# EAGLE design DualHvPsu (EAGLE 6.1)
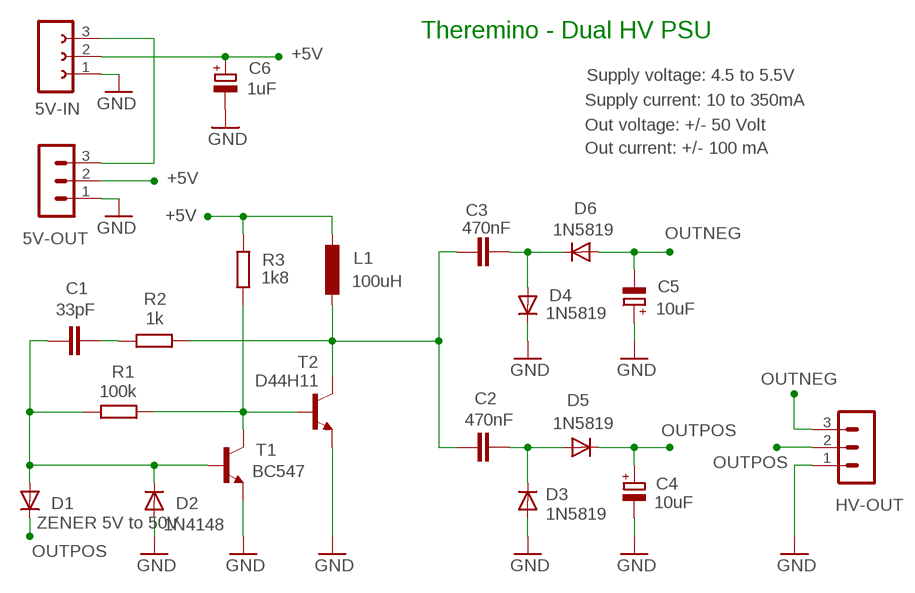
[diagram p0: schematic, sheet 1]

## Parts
5V-IN  FE03-1"  [FE03-1]
5V-OUT  MA03-1N  [MA03-1]
C1  33pF  C-EU025-024X044  [C025-024X044]
C2  470nF  C-EU050-024X044  [C050-024X044]
C3  470nF  C-EU050-024X044  [C050-024X044]
C4  10uF  CPOL-EUE2.5-5  [E2,5-5]
C5  10uF  CPOL-EUE2.5-5  [E2,5-5]
C6  1uF  CPOL-EUE2.5-5  [E2,5-5]
D1  ZENER 5V to 50V  DIODE-DO34-7  [DO34-7]
D2  1N4148  DIODE-DO34-7  [DO34-7]
D3  1N5819  DIODE-DO34-7  [DO34-7]
D4  1N5819  DIODE-DO34-7  [DO34-7]
D5  1N5819  DIODE-DO34-7  [DO34-7]
D6  1N5819  DIODE-DO34-7  [DO34-7]
HV-OUT  MA03-1N  [MA03-1]
L1  100uH  INDUCTORL_VERT_508  [L_VERT_508]
R1  100k  R-EU_0204/7  [0204/7]
R2  1k  R-EU_0204/7  [0204/7]
R3  1k8  R-EU_0204/7  [0204/7]
T1  BC547  -NPN-TO92-CBE  [TO92-CBE]
T2  D44H11  -NPN-TO220  [TO220]

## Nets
+5V: 5V-IN.2 5V-OUT.2 C6.+ L1.+ R3.2
GND: 5V-IN.1 5V-OUT.1 C4.- C5.+ C6.- D2.A D3.A D4.C HV-OUT.1 T1.E T2.3(E)
N$1: C1.1 D1.A D2.C R1.2 T1.B
N$2: C1.2 R2.2
N$3: 5V-IN.3 5V-OUT.3
N$4: C2.1 D3.C D5.A
N$5: C3.2 D4.A D6.C
N$12: C2.2 C3.1 L1.- R2.1 T2.2(C)
N$26: R1.1 R3.1 T1.C T2.1(B)
OUTNEG: C5.- D6.A HV-OUT.3
OUTPOS: C4.+ D1.C D5.C HV-OUT.2

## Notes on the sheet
- Theremino - Dual HV PSU
- Supply voltage: 4.5 to 5.5V
- Supply current: 10 to 350mA
- Out voltage: +/- 50 Volt
- Out current: +/- 100 mA

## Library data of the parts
5V-IN = 02-con-lsta-F:FE03-1: FEMALE HEADER
5V-OUT HV-OUT = 03-con-lstb-M:MA03-1: PIN HEADER
C1-C3 = 00-LIVIO:C-EU: CAPACITOR, European symbol
C4-C6 = 00-LIVIO:CPOL-EU: POLARIZED CAPACITOR, European symbol
D1-D6 = 00-LIVIO:DIODE-: DIODE
L1 = 00-LIVIO:INDUCTOR
R1-R3 = 00-LIVIO:R-EU_: RESISTOR, European symbol
T1 T2 = 00-LIVIO:*-NPN-: NPN Transistror

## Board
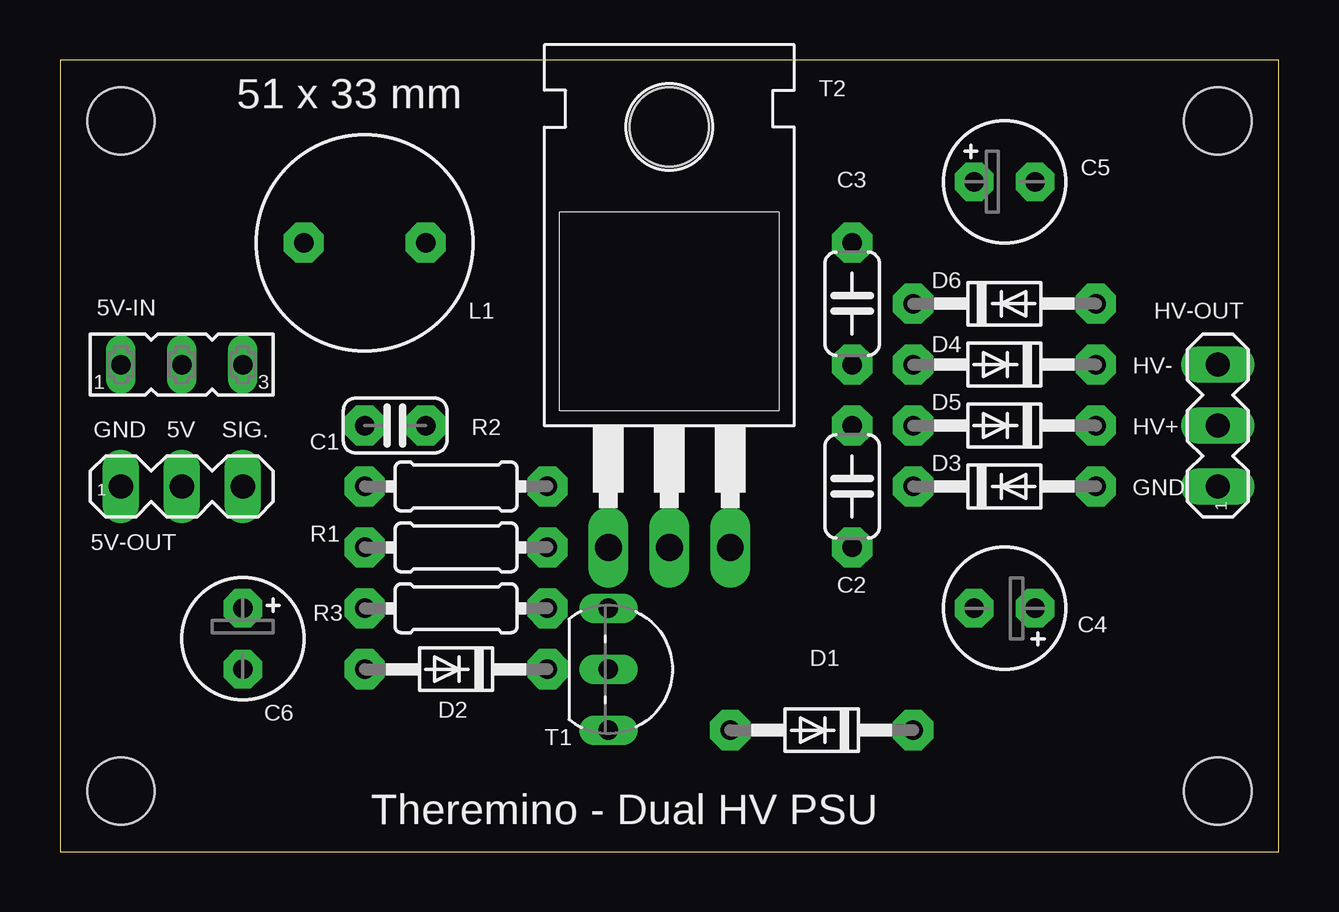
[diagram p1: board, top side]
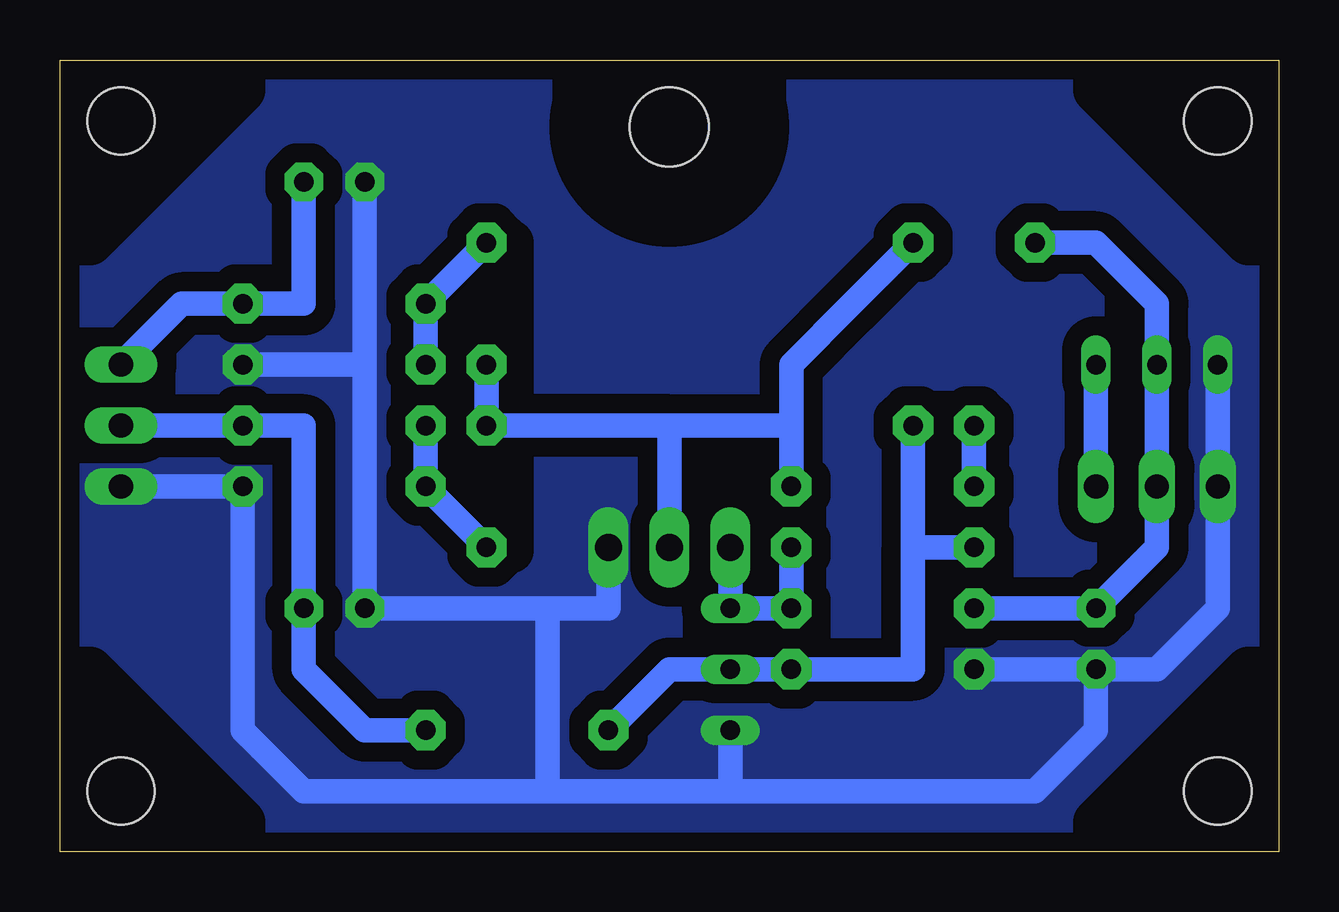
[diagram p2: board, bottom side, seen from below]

Size 50.8 x 33.02 mm. Coordinates in mm from the lower left corner, seen from the top.
Outline: 50.8,33.02 0,33.02 0,0 50.8,0 50.8,33.02
Copper layers (1*16): Top 0.035mm / dielectric 1.5mm / Bottom 0.035mm
Design rules: minimum track width 10mil, minimum drill 0.6mm, track to track 8mil, track to pad 8mil, pad to pad 8mil, via to via 8mil, smd to smd 8mil, copper to edge 31mil, drill to drill 8mil, minimum pad ring 5mil, minimum via ring 8mil, stop-mask expansion 4mil, vias tented up to drill 0mil, thermal gap 41mil
Holes 2.8 mm at 2.54,30.48 48.26,30.48 2.54,2.54 48.26,2.54
bRestrict: 10 lines

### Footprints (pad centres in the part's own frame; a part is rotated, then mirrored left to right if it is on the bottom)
FE03-1 = drill 0.813 long: 1 -2.54,0; 2 0,0; 3 2.54,0
MA03-1 = drill 1.016 long: 1 -2.54,0; 2 0,0; 3 2.54,0
C025-024X044 = drill 0.813 pad 1.676 octagon: 1 -1.27,0; 2 1.27,0
C050-024X044 = drill 0.813 pad 1.676 octagon: 1 -2.54,0; 2 2.54,0
E2,5-5 = drill 0.813 pad 1.6 octagon: + -1.27,0; - 1.27,0
DO34-7 = drill 0.813 pad 1.676 octagon: A 3.81,0; C -3.81,0
L_VERT_508 = drill 0.813 pad 1.676 octagon: + -2.54,0; - 2.54,0
0204/7 = drill 0.813 pad 1.676 octagon: 1 -3.81,0; 2 3.81,0
TO92-CBE = drill 0.813 long: B 0,0; C -2.54,0; E 2.54,0
TO220 = drill 1.118 long: 1 -2.54,-6.35; 2 0,-6.35; 3 2.54,-6.35 | hole 3.302: 0,11.176

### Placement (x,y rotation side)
5V-IN  5.08,20.32 0 top
5V-OUT  5.08,15.24 0 top
C1  13.97,17.78 180 top
C2  33.02,15.24 90 top
C3  33.02,22.86 90 top
C4  39.37,10.16 180 top
C5  39.37,27.94 0 top
C6  7.62,8.89 270 top
D1  31.75,5.08 180 top
D2  16.51,7.62 180 top
D3  39.37,15.24 0 top
D4  39.37,20.32 180 top
D5  39.37,17.78 180 top
D6  39.37,22.86 0 top
HV-OUT  48.26,17.78 90 top
L1  12.7,25.4 0 top
R1  16.51,12.7 180 top
R2  16.51,15.24 180 top
R3  16.51,10.16 180 top
T1  22.86,7.62 270 top
T2  25.4,19.05 0 top

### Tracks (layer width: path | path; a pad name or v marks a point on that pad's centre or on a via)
+5V
  Bottom 1.016: 5V-IN.2 5V-OUT.2 | 5V-OUT.2 5V-IN.2 | 5V-IN.2 5.08,22.86 7.62,25.4 L1.+ | R3.2 C6.+ 5.08,12.7 5V-OUT.2
GND
  Bottom 1.016: 22.86,2.54 20.32,2.54 15.24,2.54 10.16,2.54 7.62,5.08 C6.- | 22.86,2.54 30.48,2.54 | 30.48,2.54 40.64,2.54 43.18,5.08 D3.A HV-OUT.1 | T2.3 27.94,10.16 30.48,10.16 | 30.48,10.16 30.48,2.54 | T1.E 22.86,2.54 | 30.48,10.16 C4.- 38.1,20.32 | C6.- D2.A C6.- | C6.- 5.08,7.62 2.54,10.16 5V-IN.1 5V-OUT.1 | D4.C 38.1,20.32 | 38.1,20.32 C5.+
  pour Bottom (isolate 0.8, rank 6, no thermals): -1,-1 51.8,-1 51.8,34.02 -1,34.02
N$1
  Bottom 1.016: D1.A 25.4,7.62 T1.B D2.C 15.24,7.62 15.24,12.7 | R1.2 15.24,12.7 | C1.1 15.24,12.7
N$2
  Bottom 1.016: R2.2 C1.2
N$3
  Bottom 1.016: 5V-IN.3 5V-OUT.3
N$4
  Bottom 1.016: C2.1 D3.C D5.A
N$5
  Bottom 1.016: D4.A D6.C C3.2
N$12
  Bottom 1.016: C3.1 C2.2 25.4,17.78 | T2.2 25.4,17.78 | L1.- 17.78,22.86 20.32,20.32 20.32,17.78 | 25.4,17.78 20.32,17.78 | R2.1 20.32,17.78
N$26
  Bottom 1.016: T2.1 T1.C R3.1 | R3.1 R1.1 R3.1
OUTNEG
  Bottom 1.016: HV-OUT.3 45.72,22.86 D6.A 40.64,22.86 C5.-
OUTPOS
  Bottom 1.016: D1.C 38.1,5.08 40.64,7.62 C4.+ 40.64,17.78 D5.C HV-OUT.2

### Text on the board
tNames: 51 x 33 mm | HV- | GND | 5V | SIG. | HV+ | GND | Theremino - Dual HV PSU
